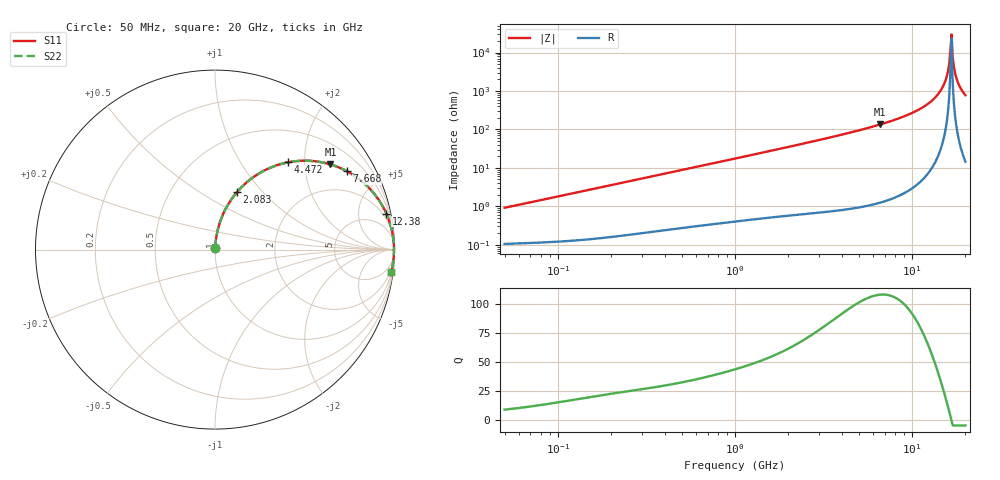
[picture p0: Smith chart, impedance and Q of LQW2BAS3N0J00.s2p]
!Murata Part Number: LQW2BAS3N0J00
!These Parameters are Measured in Series Mode Connection
!  o--[Z]--o
!Port1  Port2
!  o-------o
!Freq. Start=50[MHz] Stop=20[GHz], 401[Steps]
# Hz S RI R 50
!Freq.(Hz) S11(Real) S11(Imag) S21(Real) S21(Imag) S12(Real) S12(Imag) S22(Real) S22(Imag)
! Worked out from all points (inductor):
!   401 points, 50 MHz to 20 GHz, reference 50 ohm
!   read as one part in series: L = 2.89 nH near 51.52 MHz
!   highest Q = 108 at 6.602 GHz (marker M1), where L = 3.24 nH
!   self-resonance near 16.46 GHz
!   S11 on the Smith chart (normalised r, x): 50 MHz: 1.00, +0.02; 2.083 GHz: 1.01, +0.73; 4.472 GHz: 1.02, +1.66; 7.668 GHz: 1.03, +3.34; 12.38 GHz: 1.15, +9.51; 20 GHz: 1, -16
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5e7  0.00113 0.00912  0.9989 -0.00912  0.9989 -0.00912  0.00113 0.00912
1.364002e8  0.00193 0.0244  0.9981 -0.0244  0.9981 -0.0244  0.00193 0.0244
3.721004e8  0.00657 0.0652  0.9934 -0.0652  0.9934 -0.0652  0.00657 0.0652
1e9  0.0333 0.1682  0.9667 -0.1682  0.9667 -0.1682  0.0333 0.1682
2.083303e9  0.1217 0.3191  0.8783 -0.3191  0.8783 -0.3191  0.1217 0.3191
2.728004e9  0.1925 0.3875  0.8075 -0.3875  0.8075 -0.3875  0.1925 0.3875
4.472136e9  0.4081 0.4863  0.5919 -0.4863  0.5919 -0.4863  0.4081 0.4863
6.601595e9  0.643 0.4745  0.357 -0.4745  0.357 -0.4745  0.643 0.4745
7.442007e9  0.7166 0.446  0.2834 -0.446  0.2834 -0.446  0.7166 0.446
7.668323e9  0.7345 0.4369  0.2655 -0.4369  0.2655 -0.4369  0.7345 0.4369
1.004137e10  0.8774 0.3226  0.1226 -0.3226  0.1226 -0.3226  0.8774 0.3226
1.238412e10  0.9547 0.2002  0.0453 -0.2002  0.0453 -0.2002  0.9547 0.2002
1.396067e10  0.982 0.1216  0.018 -0.1216  0.018 -0.1216  0.982 0.1216
1.504638e10  0.9922 0.0706  0.00784 -0.0706  0.00784 -0.0706  0.9922 0.0706
1.573793e10  0.9957 0.0395  0.0043 -0.0395  0.0043 -0.0395  0.9957 0.0395
1.621653e10  0.997 0.0187  0.00303 -0.0187  0.00303 -0.0187  0.997 0.0187
1.670968e10  0.9974 -0.0021  0.00264 0.0021  0.00264 0.0021  0.9974 -0.0021
1.696185e10  0.9972 -0.0125  0.00277 0.0125  0.00277 0.0125  0.9972 -0.0125
1.747767e10  0.9963 -0.0333  0.00368 0.0333  0.00368 0.0333  0.9963 -0.0333
1.800918e10  0.9945 -0.0541  0.00547 0.0541  0.00547 0.0541  0.9945 -0.0541
1.88369e10  0.9902 -0.0851  0.00977 0.0851  0.00977 0.0851  0.9902 -0.0851
2e10  0.9815 -0.1258  0.0185 0.1258  0.0185 0.1258  0.9815 -0.1258
